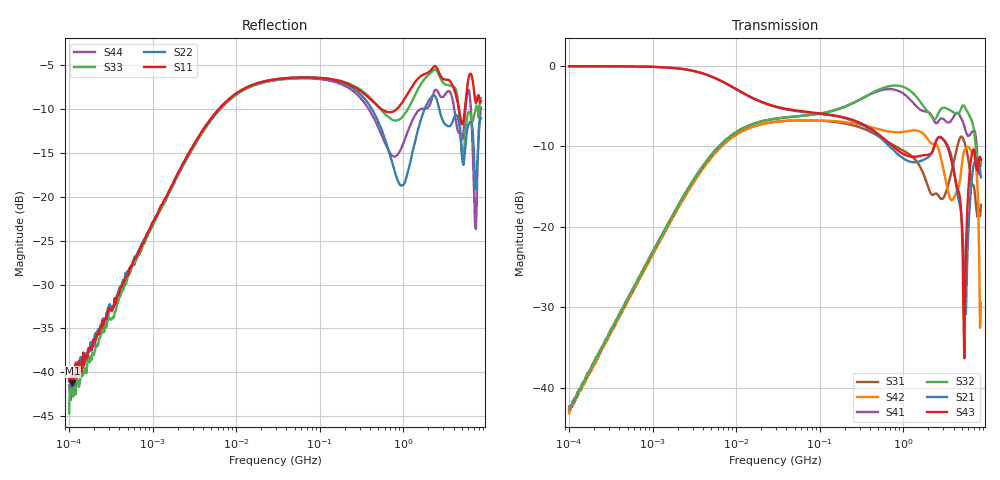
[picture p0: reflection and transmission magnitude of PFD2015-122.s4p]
# MHz S MA R 50
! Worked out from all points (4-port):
!   498 points, 100 kHz to 8.5 GHz, reference 50 ohm
!   strongest paths, dB at 100 kHz, 1.698 MHz, 29.49 MHz, 500.7 MHz, 8.5 GHz:
!     S43: -0.1, -0.3, -5.1, -8.5, -11.6
!     S21: -0.1, -0.3, -5.2, -8.7, -13.9
!     S32: -42.6, -18.8, -6.6, -3.0, -12.4
!     S41: -42.3, -18.8, -6.6, -3.2, -11.6
!     S42: -43.2, -19.1, -7.0, -7.9, -29.5
!     S31: -42.9, -19.1, -7.0, -8.7, -17.3
!   lowest |S11| = -41.3 dB at 109.6 kHz (marker M1), VSWR 1.02, Z = 50.5 + j0.74 ohm
!   |S11| at or under -10 dB: start of sweep to 6.197 MHz; 546.8 MHz to 837 MHz (290.2 MHz wide, 41.9 % of centre); 4.64 GHz to 5.469 GHz (829.5 MHz wide, 16.4 % of centre)
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0.1  0.009201 59.4  0.9906 -0.4  0.007183 -90.2  0.007657 88.2
     0.9906 -0.4  0.008874 69.1  0.007447 91.6  0.006928 -93.1
     0.007183 -90.2  0.007447 91.6  0.005842 39.9  0.9902 -0.4
     0.007657 88.2  0.006928 -93.1  0.9902 -0.4  0.008421 64.0
0.1095654  0.008639 58.0  0.9895 -0.5  0.007817 -92.4  0.008062 88.2
           0.9895 -0.5  0.009345 54.1  0.008195 88.4  0.007642 -91.2
           0.007817 -92.4  0.008195 88.4  0.007978 43.5  0.9893 -0.4
           0.008062 88.2  0.007642 -91.2  0.9893 -0.4  0.009486 61.9
19.10821  0.4482 16.8  0.5971 -20.7  0.4296 -164.9  0.4473 19.5
          0.5971 -20.7  0.4482 15.8  0.4472 19.6  0.4292 -165.9
          0.4296 -164.9  0.4472 19.6  0.4427 17.2  0.6017 -20.7
          0.4473 19.5  0.4292 -165.9  0.6017 -20.7  0.4423 16.3
389.4413  0.3659 -63.3  0.4038 -105.5  0.3914 79.2  0.6573 -41.1
          0.4038 -105.5  0.3359 -85.1  0.6599 -38.8  0.4176 62.7
          0.3914 79.2  0.6599 -38.8  0.372 -65.9  0.4118 -106.4
          0.6573 -41.1  0.4176 62.7  0.4118 -106.4  0.3142 -80.4
1219.999  0.4105 -151.2  0.2523 63.6  0.2775 -102.0  0.6117 -171.3
          0.2523 63.6  0.1588 -143.1  0.6952 -170.4  0.3934 -122.5
          0.2775 -102.0  0.6952 -170.4  0.3372 -154.1  0.2721 57.8
          0.6117 -171.3  0.3934 -122.5  0.2721 57.8  0.2574 -148.4
5383.342  0.2949 -16.4  0.04845 -30.8  0.3362 77.9  0.4206 14.2
          0.04845 -30.8  0.1656 -10.5  0.5604 9.0  0.2957 80.7
          0.3362 77.9  0.5604 9.0  0.1921 -38.4  0.01523 92.9
          0.4206 14.2  0.2957 80.7  0.01523 92.9  0.265 -23.2
8500  0.3503 -52.8  0.2023 11.4  0.1365 50.5  0.2627 -6.4
      0.2023 11.4  0.2795 -34.8  0.2393 -41.6  0.03367 115.9
      0.1365 50.5  0.2393 -41.6  0.3648 -73.1  0.2617 9.9
      0.2627 -6.4  0.03367 115.9  0.2617 9.9  0.3225 -41.2
